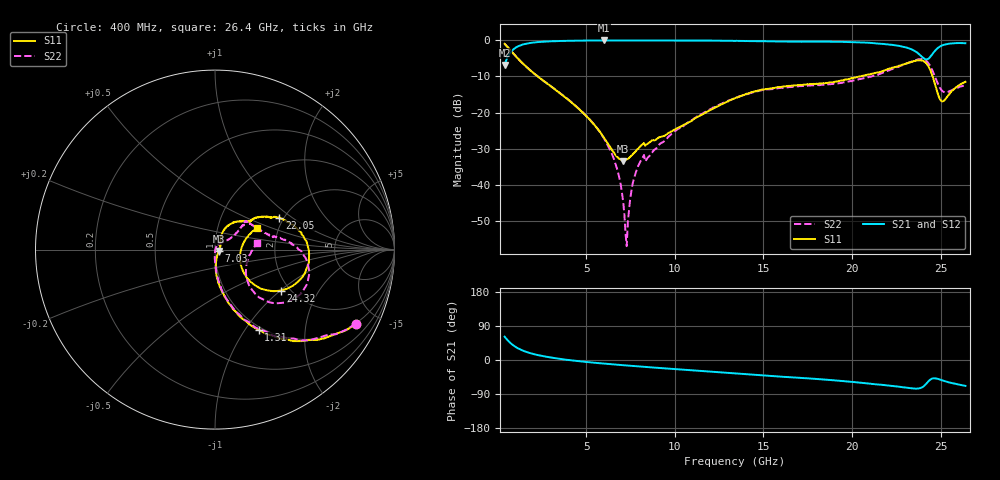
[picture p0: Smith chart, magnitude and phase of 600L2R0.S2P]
!  American Technical Ceramics  Date:  6/18/2004
!  One Norden Lane
!  Huntington Station,  NY.  11746-2102
!  Tel:  (631) 622-4700  Fax:  (631) 622-4748
!  Part Number  600L2R0  Mounting Orientation: Vertical
!  Description: Ultra Low ESR Microwave capacitors
!  Application: Coupling, Bypass, Tuning, DC Block
!  Filters, Matching
# GHZ S DB R 50
! Freq  |S11|  S11 Ph  |S21|  S21 Ph  |S12|  S12 Ph  |S22|  S22 Ph
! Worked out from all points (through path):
!   401 points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, 400 MHz to 26.4 GHz, reference 50 ohm
!   highest |S21| = -0.11 dB at 5.99 GHz (marker M1); lowest = -6.9 dB at 400 MHz (marker M2)
!   group delay of S21, straight-line fit = 10.1 ps
!   lowest |S11| = -33.4 dB at 7.095 GHz (marker M3), VSWR 1.04, Z = 52.1 - j0.717 ohm
!   |S11| at or under -10 dB: 2.266 GHz to 20.47 GHz (18.2 GHz wide, 160 % of centre); 24.55 GHz to end of sweep
!   |S22| runs from -56.8 to -1.1 dB; largest |S21 - S12| = 0.0076
!   S11 on the Smith chart (normalised r, x): 400 MHz: 0.97, -3.78; 1.31 GHz: 0.96, -1.16; 7.03 GHz: 1.04, -0.02; 22.05 GHz: 1.89, +0.80; 24.32 GHz: 1.79, -1.01; 26.4 GHz: 1.56, +0.40
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0.4  -1.04 -28.0  -6.89 61.5  -6.90 61.4  -1.05 -27.8
1.31  -5.87 -61.4  -1.42 27.2  -1.44 27.3  -5.92 -61.2
2.415  -10.57 -76.5  -0.51 11.5  -0.51 11.5  -10.61 -75.8
4.755  -19.76 -87.9  -0.15 -3.9  -0.15 -3.9  -19.62 -87.2
5.99  -26.78 -78.4  -0.11 -9.5  -0.12 -9.5  -26.96 -91.3
6.64  -31.55 -52.0  -0.12 -12.0  -0.12 -12.1  -33.86 -91.2
7.03  -33.20 -23.8  -0.12 -13.5  -0.12 -13.5  -42.39 -85.9
7.095  -33.39 -18.8  -0.12 -13.8  -0.12 -13.8  -44.76 -81.6
7.16  -33.28 -13.8  -0.12 -14.0  -0.13 -14.0  -48.19 -74.7
7.29  -32.86 -3.3  -0.11 -14.5  -0.12 -14.5  -56.81 10.2
7.615  -31.58 15.3  -0.12 -15.7  -0.12 -15.7  -39.77 66.4
7.94  -29.94 28.5  -0.12 -16.9  -0.12 -16.8  -34.70 67.4
9.11  -26.81 47.1  -0.13 -21.0  -0.13 -20.9  -28.86 56.5
13.4  -16.05 60.2  -0.23 -35.5  -0.21 -35.4  -15.98 38.3
17.755  -12.12 39.3  -0.43 -49.4  -0.43 -49.3  -12.46 40.5
22.045  -7.96 26.5  -1.22 -67.2  -1.21 -67.0  -8.44 9.1
22.11  -7.85 25.8  -1.25 -67.6  -1.25 -67.7  -8.30 8.2
23.735  -5.59 -3.1  -3.67 -75.3  -3.65 -75.1  -5.32 -13.9
24.32  -7.31 -32.0  -5.14 -55.9  -5.11 -55.9  -6.44 -38.5
24.71  -12.57 -41.4  -2.82 -48.5  -2.82 -48.5  -10.42 -47.3
25.1  -16.94 -8.2  -1.46 -53.9  -1.46 -53.8  -14.04 -29.2
26.4  -11.51 27.0  -0.87 -68.2  -0.87 -68.2  -12.48 9.1
